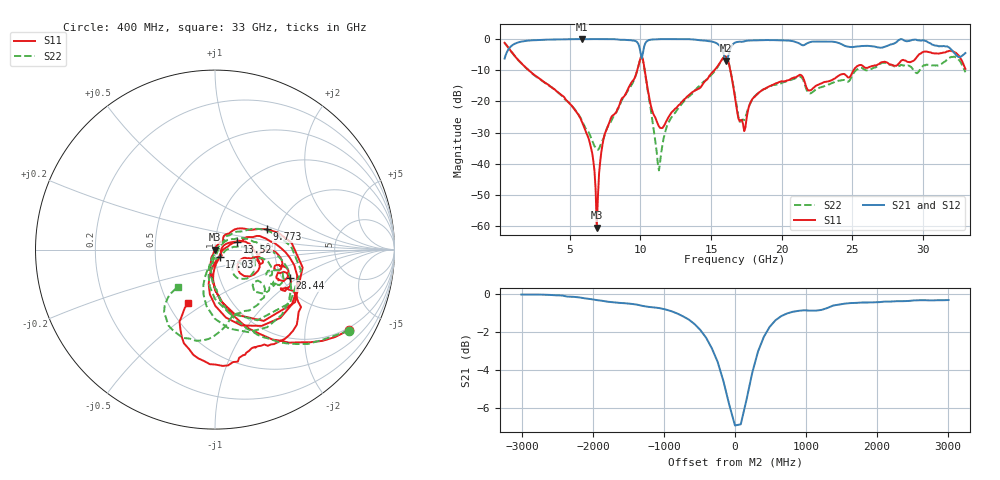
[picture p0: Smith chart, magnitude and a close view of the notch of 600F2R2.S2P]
!  American Technical Ceramics  Date:  11/23/05
!  One Norden Lane
!  Huntington Station,  NY.  11746-2102
!  Tel:  (631) 622-4700  Fax:  (631) 622-4748
!  Part Number  600F2R2  Mounting Orientation: Horizontal
!  Description: Ultra Low ESR Microwave capacitors
!  Application: Coupling, Bypass, Tuning, DC Block
!  Filters, Matching
# GHZ S DB R 50
! Freq  |S11|  S11 Ph  |S21|  S21 Ph  |S12|  S12 Ph  |S22|  S22 Ph
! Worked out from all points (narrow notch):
!   401 points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, 400 MHz to 33 GHz, reference 50 ohm
!   highest |S21| = 0.00 dB at 5.861 GHz (marker M1); lowest = -6.9 dB at 16.05 GHz (marker M2)
!   notch at M2: 6.4 dB deep, 505 MHz wide at half that depth
!   lowest |S11| = -60.5 dB at 6.92 GHz (marker M3), VSWR 1.00, Z = 49.9 - j0.0422 ohm
!   |S11| at or under -10 dB: 2.107 GHz to 9.783 GHz (7.676 GHz wide, 129 % of centre); 10.31 GHz to 15.24 GHz (4.927 GHz wide, 38.6 % of centre); 16.37 GHz to 25.09 GHz (8.717 GHz wide, 42.1 % of centre)
!   |S22| runs from -42.1 to -1.2 dB; largest |S21 - S12| = 0.014
!   S11 on the Smith chart (normalised r, x): 400 MHz: 0.91, -3.38; 9.773 GHz: 1.74, +0.44; 13.52 GHz: 1.28, +0.11; 17.03 GHz: 1.05, -0.09; 28.44 GHz: 2.20, -0.86; 33 GHz: 0.63, -0.42
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0.4  -1.20 -30.9  -6.24 58.9  -6.24 58.8  -1.19 -31.2
1.949  -9.35 -78.0  -0.56 11.2  -0.57 10.9  -9.43 -79.1
5.861  -26.44 -114.5  0.00 -21.2  -0.01 -21.2  -26.07 -96.9
6.513  -34.87 -113.4  -0.01 -25.2  -0.02 -25.2  -31.58 -71.4
6.92  -60.46 -153.6  -0.01 -27.8  0.00 -27.9  -35.41 -31.9
7.572  -29.45 57.7  -0.01 -32.1  0.00 -32.3  -29.43 32.0
9.773  -10.17 21.4  -0.97 -54.9  -0.98 -54.7  -10.26 20.6
10.262  -8.45 -72.9  -2.56 -23.1  -2.58 -23.7  -8.80 -77.3
11.321  -28.03 -47.4  0.00 -45.3  0.00 -45.2  -42.11 -22.0
12.055  -24.61 9.2  -0.01 -51.8  -0.01 -51.9  -26.29 41.4
13.522  -17.65 19.4  -0.05 -63.3  -0.05 -63.3  -18.13 28.3
15.315  -9.56 6.5  -1.16 -80.5  -1.14 -80.4  -10.07 -1.4
16.048  -5.57 -46.3  -6.92 -75.0  -6.78 -74.8  -5.66 -56.1
16.7  -18.80 -100.3  -1.15 -58.4  -1.18 -58.5  -18.00 -110.3
17.026  -26.28 -57.6  -0.84 -64.7  -0.85 -64.8  -26.49 -69.0
19.308  -14.79 12.4  -0.33 -83.9  -0.36 -83.8  -14.88 2.4
22.161  -16.05 -19.4  -0.81 -96.2  -0.84 -96.3  -17.10 -31.7
27.621  -8.10 -25.4  -1.93 -117.1  -1.89 -116.7  -8.19 -29.5
28.436  -7.02 -20.6  -0.01 -127.0  -0.01 -126.5  -8.27 -30.0
29.903  -4.39 -40.2  -0.43 -147.8  -0.40 -147.3  -9.03 -38.0
31.941  -3.75 -86.3  -3.05 -171.1  -3.04 -170.5  -5.84 -97.8
33  -9.56 -116.5  -4.47 -153.8  -4.44 -153.9  -10.64 -134.8
